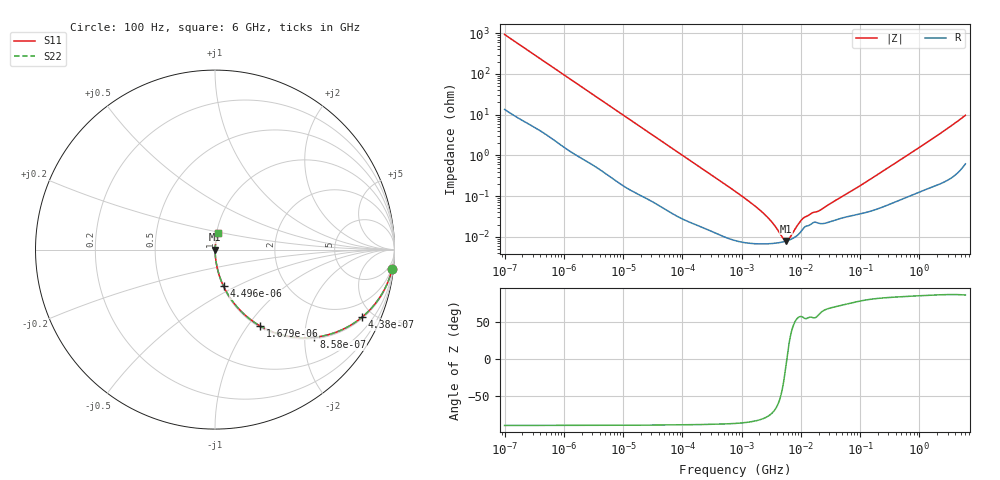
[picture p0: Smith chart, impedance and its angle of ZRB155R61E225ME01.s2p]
!Murata Part Number: ZRB155R61E225ME01
!These Parameters are Measured in Series Mode Connection
!Data Generated on Jun 10, 2025
!  o--ll--o
!Port1  Port2
!  o------o
!Operation Temp=25[degC], DC Bias Voltage=0[V]
!Freq. Start=100[Hz] Stop=6[GHz] 401[Steps]
# Hz S RI R 50
!Freq.(Hz) S11(Real) S11(Imag) S21(Real) S21(Imag) S12(Real) S12(Imag) S22(Real) S22(Imag)
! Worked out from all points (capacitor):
!   401 points, 100 Hz to 6 GHz, reference 50 ohm
!   read as one part in series: C = 1.7 uF near 109 Hz
!   lowest |Z| = 8 mohm at 5.555 MHz (marker M1)
!   series resonance near 5.795 MHz, so ESL is about 440 pH
!   S11 on the Smith chart (normalised r, x): 100 Hz: 1, -19; 438 Hz: 1.07, -4.32; 858 Hz: 1.04, -2.22; 1.679 kHz: 1.02, -1.14; 4.496 kHz: 1.01, -0.43; 6 GHz: 1.01, +0.19
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100  0.9871 -0.1057  0.0129 0.1057  0.0129 0.1057  0.9871 -0.1057
245  0.9332 -0.2419  0.0668 0.2419  0.0668 0.2419  0.9332 -0.2419
438  0.8194 -0.3762  0.1806 0.3762  0.1806 0.3762  0.8194 -0.3762
858  0.5522 -0.4889  0.4478 0.4889  0.4478 0.4889  0.5522 -0.4889
1174  0.4011 -0.4819  0.5989 0.4819  0.5989 0.4819  0.4011 -0.4819
1679  0.2502 -0.4247  0.7498 0.4247  0.7498 0.4247  0.2502 -0.4247
2008  0.1909 -0.3843  0.8091 0.3843  0.8091 0.3843  0.1909 -0.3843
4496  0.0481 -0.2049  0.9519 0.2049  0.9519 0.2049  0.0481 -0.2049
11514  0.00876 -0.0844  0.9912 0.0844  0.9912 0.0844  0.00876 -0.0844
40335  0.0012 -0.0247  0.9988 0.0247  0.9988 0.0247  0.0012 -0.0247
774597  8.31e-05 -0.00132  0.9999 0.00132  0.9999 0.00132  8.31e-05 -0.00132
2268635  6.74e-05 -0.000391  0.9999 0.000391  0.9999 0.000391  6.74e-05 -0.000391
3245845  6.87e-05 -0.000222  0.9999 0.000222  0.9999 0.000222  6.87e-05 -0.000222
4643984  7.37e-05 -8.1e-05  0.9999 8.1e-05  0.9999 8.1e-05  7.37e-05 -8.1e-05
5554849  7.85e-05 -1.54e-05  0.9999 1.54e-05  0.9999 1.54e-05  7.85e-05 -1.54e-05
6644369  8.59e-05 5.01e-05  0.9999 -5.01e-05  0.9999 -5.01e-05  8.59e-05 5.01e-05
1.039699e7  0.000144 0.000224  0.9999 -0.000224  0.9999 -0.000224  0.000144 0.000224
1.555665e7  0.000216 0.000323  0.9998 -0.000323  0.9998 -0.000323  0.000216 0.000323
2.225763e7  0.000211 0.000422  0.9998 -0.000422  0.9998 -0.000422  0.000211 0.000422
3.124326e8  0.000655 0.00518  0.9993 -0.00518  0.9993 -0.00518  0.000655 0.00518
1.95892e9  0.00274 0.0299  0.9973 -0.0299  0.9973 -0.0299  0.00274 0.0299
6e9  0.0152 0.0944  0.9848 -0.0944  0.9848 -0.0944  0.0152 0.0944
